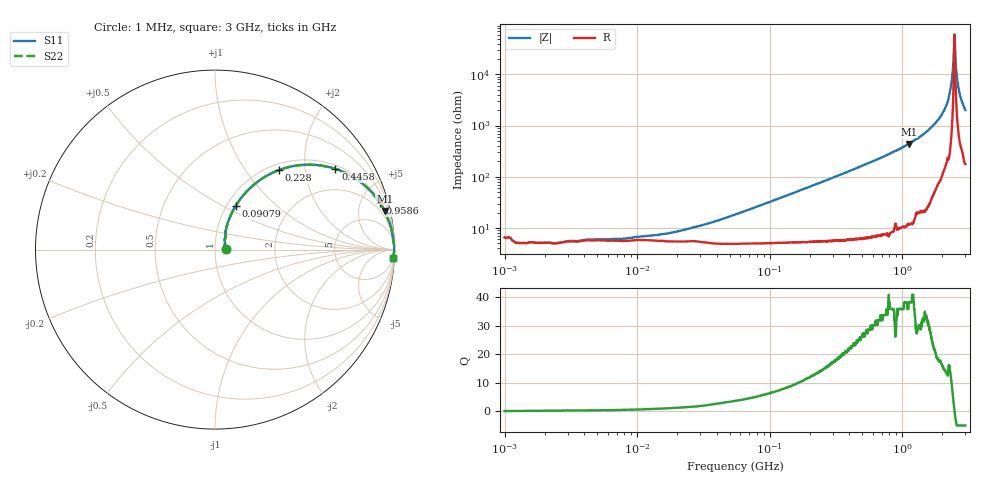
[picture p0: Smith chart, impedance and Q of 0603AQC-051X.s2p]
!s-Parameter Generated by FASTRON Sdn. Bhd.
!FASTRON P/N : 0603AQC-051X
!Keysight Technologies: E4991B_MY54100416_A.01.15
!Date: Thu Jun 25 13:54:37 2026
!Version  :Rev00  Thu Jun 25 13:54:37 2026
!Data & Calibration Information:
!Freq  S11  S21  S12  S22
!PortZ  Port1:50+j0  Port2:50+j0
!When reading reference impedance value at option line is always used.
! Remarks : This data is being provided solely for informational purposes.
# Hz S dB R 50
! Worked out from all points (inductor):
!   1601 points, 1 MHz to 3 GHz, reference 50 ohm
!   read as one part in series: L = 51.1 nH near 45.74 MHz
!   highest Q = 38.2 at 1.119 GHz (marker M1), where L = 62.3 nH
!   self-resonance near 2.481 GHz
!   S11 on the Smith chart (normalised r, x): 1 MHz: 1.13, +0.01; 90.79 MHz: 1.10, +0.58; 228 MHz: 1.11, +1.45; 445.8 MHz: 1.12, +2.90; 958.6 MHz: 1.19, +7.05; 3 GHz: 5, -40
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1000000  -24.20 2.8  -0.55 -0.2  -0.55 -0.2  -24.20 2.8
1316819  -26.30 4.9  -0.43 -0.2  -0.43 -0.2  -26.30 4.9
3804036  -25.30 12.4  -0.47 -0.7  -0.47 -0.7  -25.30 12.4
1.447069e7  -23.10 37.7  -0.49 -2.6  -0.49 -2.6  -23.10 37.7
5.504702e7  -15.30 64.9  -0.54 -9.6  -0.54 -9.6  -15.30 64.9
9.079332e7  -11.40 64.7  -0.74 -15.4  -0.74 -15.4  -11.40 64.7
2.083556e8  -5.44 53.2  -1.91 -32.2  -1.91 -32.2  -5.44 53.2
2.279937e8  -4.90 51.2  -2.15 -34.6  -2.15 -34.6  -4.90 51.2
4.457915e8  -1.86 33.8  -5.08 -53.8  -5.08 -53.8  -1.86 33.8
7.925923e8  -0.60 19.7  -9.45 -68.9  -9.45 -68.9  -0.60 19.7
9.585869e8  -0.40 15.7  -11.30 -72.7  -11.30 -72.7  -0.40 15.7
1.11944e9  -0.27 12.8  -13.10 -75.7  -13.10 -75.7  -0.27 12.8
1.565327e9  -0.10 7.0  -18.20 -81.1  -18.20 -81.1  -0.10 7.0
2.03054e9  -0.04 3.1  -25.20 -83.2  -25.20 -83.2  -0.04 3.1
2.255531e9  -0.02 1.5  -31.50 -84.8  -31.50 -84.8  -0.02 1.5
2.335937e9  -0.01 1.0  -35.50 -84.2  -35.50 -84.2  -0.01 1.0
2.41921e9  -0.01 0.4  -42.70 -78.0  -42.70 -78.0  -0.01 0.4
2.480502e9  -0.01 0.0  -55.60 -11.4  -55.60 -11.4  -0.01 0.0
2.556106e9  -0.02 -0.4  -42.10 75.6  -42.10 75.6  -0.02 -0.4
2.634014e9  -0.02 -0.9  -36.10 80.6  -36.10 80.6  -0.02 -0.9
2.714296e9  -0.03 -1.4  -32.50 82.1  -32.50 82.1  -0.03 -1.4
3e9  -0.05 -2.8  -26.10 82.1  -26.10 82.1  -0.05 -2.8
